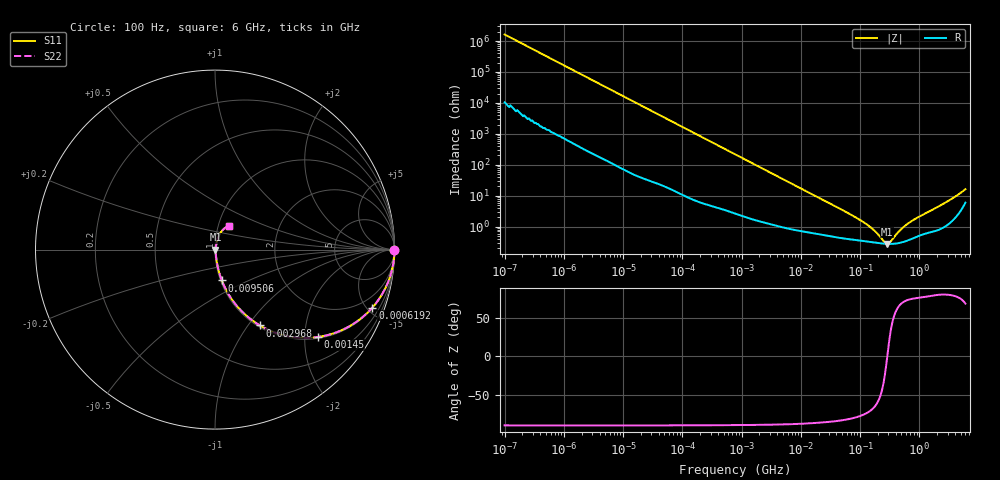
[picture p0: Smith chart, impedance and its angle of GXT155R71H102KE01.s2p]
!Murata Part Number: GXT155R71H102KE01
!These Parameters are Measured in Series Mode Connection
!Data Generated on Jan 08, 2026
!  o--ll--o
!Port1  Port2
!  o------o
!Operation Temp=25[degC], DC Bias Voltage=0[V]
!Freq. Start=100[Hz] Stop=6[GHz] 401[Steps]
# Hz S RI R 50
!Freq.(Hz) S11(Real) S11(Imag) S21(Real) S21(Imag) S12(Real) S12(Imag) S22(Real) S22(Imag)
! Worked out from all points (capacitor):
!   401 points, 100 Hz to 6 GHz, reference 50 ohm
!   read as one part in series: C = 976 pF near 109 Hz
!   lowest |Z| = 278 mohm at 285.7 MHz (marker M1)
!   series resonance near 288.1 MHz, so ESL is about 310 pH
!   S11 on the Smith chart (normalised r, x): 100 Hz: open; 619.2 kHz: 1.06, -5.41; 1.45 MHz: 1.04, -2.32; 2.968 MHz: 1.02, -1.14; 9.506 MHz: 1.01, -0.36; 6 GHz: 1.12, +0.30
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100  1 -6.14e-05  4e-07 6.14e-05  4e-07 6.14e-05  1 -6.14e-05
150  1 -9.18e-05  5e-07 9.18e-05  5e-07 9.18e-05  1 -9.18e-05
179  1 -0.00011  6e-07 0.00011  6e-07 0.00011  1 -0.00011
2008  1 -0.00122  6.7e-06 0.00122  6.7e-06 0.00122  1 -0.00122
40335  0.9993 -0.0244  0.000734 0.0244  0.000734 0.0244  0.9993 -0.0244
193316  0.9859 -0.1144  0.0141 0.1144  0.0141 0.1144  0.9859 -0.1144
619225  0.8768 -0.323  0.1232 0.323  0.1232 0.323  0.8768 -0.323
774597  0.821 -0.3773  0.179 0.3773  0.179 0.3773  0.821 -0.3773
1449809  0.573 -0.4871  0.427 0.4871  0.427 0.4871  0.573 -0.4871
2967816  0.2501 -0.4225  0.7499 0.4225  0.7499 0.4225  0.2501 -0.4225
5079039  0.1076 -0.2962  0.8924 0.2962  0.8924 0.2962  0.1076 -0.2962
9506416  0.038 -0.172  0.962 0.172  0.962 0.172  0.038 -0.172
1.555665e7  0.0181 -0.1081  0.9819 0.1081  0.9819 0.1081  0.0181 -0.1081
1.115611e8  0.00364 -0.0139  0.9964 0.0139  0.9964 0.0139  0.00364 -0.0139
1.669249e8  0.00316 -0.00743  0.9968 0.00743  0.9968 0.00743  0.00316 -0.00743
2.497637e8  0.00283 -0.00191  0.9972 0.00191  0.9972 0.00191  0.00283 -0.00191
2.856706e8  0.00278 -0.000112  0.9972 0.000112  0.9972 0.000112  0.00278 -0.000112
3.124326e8  0.00276 0.0011  0.9972 -0.0011  0.9972 -0.0011  0.00276 0.0011
4.888888e8  0.0031 0.00751  0.9969 -0.00751  0.9969 -0.00751  0.0031 0.00751
6.994765e8  0.00401 0.0134  0.996 -0.0134  0.996 -0.0134  0.00401 0.0134
3.205649e9  0.0171 0.068  0.9829 -0.068  0.9829 -0.068  0.0171 0.068
6e9  0.0753 0.1322  0.9247 -0.1322  0.9247 -0.1322  0.0753 0.1322
